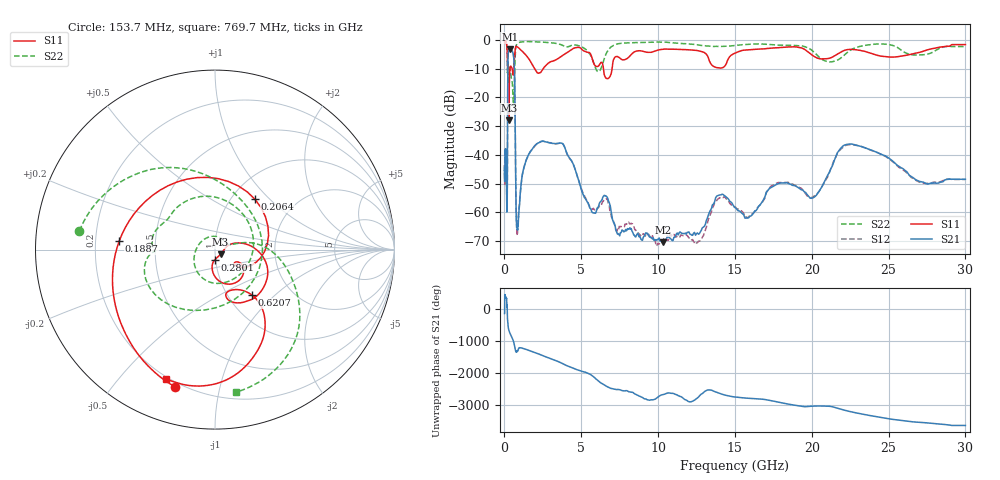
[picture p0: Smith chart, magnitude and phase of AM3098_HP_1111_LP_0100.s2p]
! Date/Time: Thu, Feb 28, 2019 8:47 AM
! Network Analyzer: Agilent Technologies E8364B Rev: A.07.50.67
! Sweep from 0.010 to 30.000 GHz, 1601 Points, Sweep Type: LOG
! Power Supply: 5.022 V, 0.002 A
# Hz S DB R 50
!freq MagS11 AngS11 MagS21 AngS21 MagS12 AngS12 MagS22 AngS22
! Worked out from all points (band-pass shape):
!   1601 points, 10 MHz to 30 GHz, reference 50 ohm
!   highest |S21| = -3.38 dB at 338.8 MHz (marker M1); lowest = -70.3 dB at 10.33 GHz (marker M2)
!   |S21| within 3 dB of the highest: 228.1 MHz to 607 MHz (378.9 MHz wide, 90.8 % of centre)
!   lowest |S11| = -27.9 dB at 290.1 MHz (marker M3), VSWR 1.08, Z = 53.1 - j2.69 ohm
!   |S11| at or under -10 dB: 210 MHz to 357.9 MHz (147.9 MHz wide, 52.1 % of centre); 1.959 GHz to 2.53 GHz (570.5 MHz wide, 25.4 % of centre); 6.44 GHz to 7.005 GHz (565.1 MHz wide, 8.41 % of centre)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
!   |S22| runs from -22.9 to -0.5 dB; largest |S21 - S12| = 0.012
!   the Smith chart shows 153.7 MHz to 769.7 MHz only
!   S11 on the Smith chart (normalised r, x): 153.7 MHz: 0.18, -0.73; 188.7 MHz: 0.30, +0.04; 206.4 MHz: 1.28, +0.82; 280.1 MHz: 0.99, -0.11; 620.7 MHz: 1.29, -0.73; 769.7 MHz: 0.19, -0.68
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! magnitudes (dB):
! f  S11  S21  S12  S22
! 10 MHz  -0.4  -45.3  -43.6  -0.5
! 38.04 MHz  -0.2  -41.2  -40.6  -0.6
! 94.1 MHz  -0.8  -39.1  -39.7  -1.1
! 144.7 MHz  -1.6  -56.3  -55.0  -1.9
! 153.7 MHz  -2.0  -59.3  -58.2  -2.4
! 188.7 MHz  -5.4  -52.0  -51.6  -9.2
! 206.4 MHz  -8.9  -21.8  -21.8  -8.9
! 227 MHz  -17.6  -6.6  -6.6  -9.2
! 280.1 MHz  -25.2  -3.7  -3.7  -9.5
! 290.1 MHz  -27.9  -3.6  -3.5  -9.8
! 338.8 MHz  -11.4  -3.4  -3.4  -10.0
! 550.5 MHz  -12.0  -4.5  -4.5  -19.6
! 620.7 MHz  -9.7  -7.4  -7.3  -20.8
! 672.5 MHz  -4.9  -16.6  -16.6  -9.4
! 769.7 MHz  -2.3  -62.3  -61.1  -1.9
! 2.084 GHz  -11.1  -36.3  -36.2  -0.7
! 3.779 GHz  -5.4  -36.1  -36.0  -1.9
! 7.926 GHz  -6.7  -66.4  -64.0  -1.1
! 10.33 GHz  -3.3  -70.3  -69.6  -0.8
! 20.1 GHz  -5.6  -54.9  -54.6  -4.1
! 22.56 GHz  -3.4  -36.2  -36.5  -3.5
! 30 GHz  -1.7  -48.5  -48.5  -2.4
